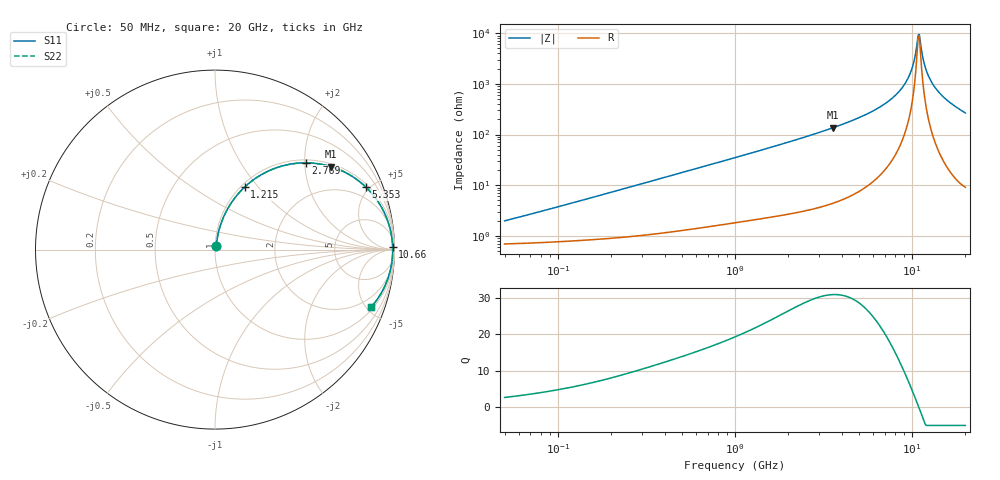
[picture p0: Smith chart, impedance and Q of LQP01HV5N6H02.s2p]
!Murata Part Number: LQP01HV5N6H02
!These Parameters are Measured in Series Mode Connection
!  o--[Z]--o
!Port1  Port2
!  o-------o
!Freq. Start=50[MHz] Stop=20[GHz], 401[Steps]
# Hz S RI R 50
!Freq.(Hz) S11(Real) S11(Imag) S21(Real) S21(Imag) S12(Real) S12(Imag) S22(Real) S22(Imag)
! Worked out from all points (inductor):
!   401 points, 50 MHz to 20 GHz, reference 50 ohm
!   read as one part in series: L = 5.88 nH near 57.22 MHz
!   highest Q = 30.9 at 3.572 GHz (marker M1), where L = 6.06 nH
!   self-resonance near 10.82 GHz
!   S11 on the Smith chart (normalised r, x): 50 MHz: 1.01, +0.04; 1.215 GHz: 1.04, +0.85; 2.769 GHz: 1.07, +2.02; 5.353 GHz: 1.17, +4.77; 10.66 GHz: open; 20 GHz: 1.18, -5.32
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5e7  0.00724 0.0183  0.9928 -0.0183  0.9928 -0.0183  0.00724 0.0183
1.364002e8  0.0105 0.0488  0.9895 -0.0488  0.9895 -0.0488  0.0105 0.0488
3.721004e8  0.0277 0.1273  0.9723 -0.1273  0.9723 -0.1273  0.0277 0.1273
1e9  0.1215 0.3018  0.8785 -0.3018  0.8785 -0.3018  0.1215 0.3018
1.214974e9  0.1647 0.3479  0.8353 -0.3479  0.8353 -0.3479  0.1647 0.3479
2.728004e9  0.4963 0.4834  0.5037 -0.4834  0.5037 -0.4834  0.4963 0.4834
2.769174e9  0.5044 0.4834  0.4956 -0.4834  0.4956 -0.4834  0.5044 0.4834
3.572216e9  0.6448 0.4627  0.3552 -0.4627  0.3552 -0.4627  0.6448 0.4627
5.352748e9  0.8419 0.3471  0.1581 -0.3471  0.1581 -0.3471  0.8419 0.3471
7.442007e9  0.9465 0.1991  0.0535 -0.1991  0.0535 -0.1991  0.9465 0.1991
8.516016e9  0.9715 0.1309  0.0285 -0.1309  0.0285 -0.1309  0.9715 0.1309
9.457416e9  0.9837 0.0762  0.0163 -0.0762  0.0163 -0.0762  0.9837 0.0762
1.004137e10  0.9879 0.0445  0.0121 -0.0445  0.0121 -0.0445  0.9879 0.0445
1.066139e10  0.9899 0.0126  0.0101 -0.0126  0.0101 -0.0126  0.9899 0.0126
1.082228e10  0.9901 0.00455  0.00993 -0.00455  0.00993 -0.00455  0.9901 0.00455
1.115139e10  0.99 -0.0115  0.00997 0.0115  0.00997 0.0115  0.99 -0.0115
1.166392e10  0.989 -0.0357  0.011 0.0357  0.011 0.0357  0.989 -0.0357
1.201863e10  0.9876 -0.0518  0.0124 0.0518  0.0124 0.0518  0.9876 -0.0518
1.257102e10  0.9845 -0.076  0.0155 0.076  0.0155 0.076  0.9845 -0.076
1.354865e10  0.9765 -0.1162  0.0235 0.1162  0.0235 0.1162  0.9765 -0.1162
1.597544e10  0.946 -0.2043  0.054 0.2043  0.054 0.2043  0.946 -0.2043
2e10  0.8682 -0.3216  0.1318 0.3216  0.1318 0.3216  0.8682 -0.3216
